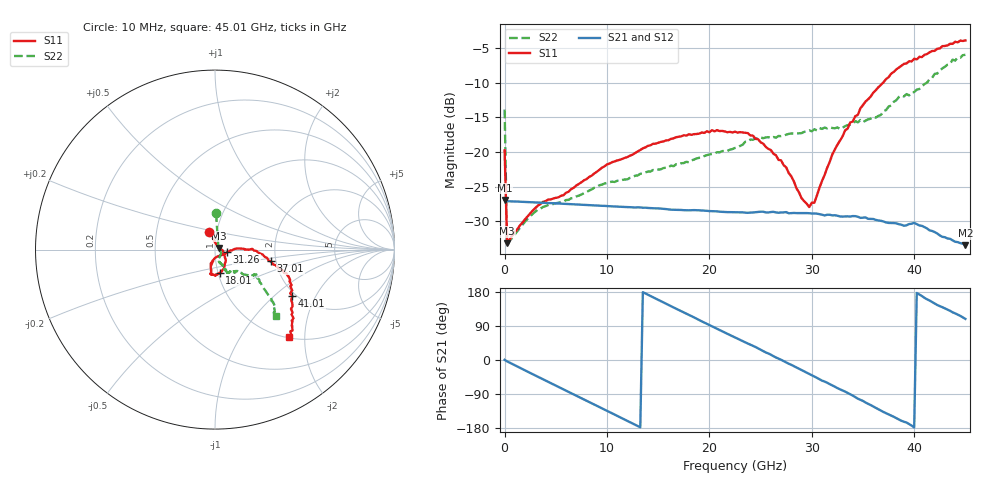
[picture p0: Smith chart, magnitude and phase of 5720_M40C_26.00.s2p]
! Device:  ADRF5720
! Description: 0.5dB LSB GaAs MMIC 6-bit Digital Attenuator
! Frequency:  0.000009 -  40 GHz
! Ports:
!	RF1	= Port 1
!	RF2	= Port 2
! Vdd:  3.3 Volt
! Vss:  -3.3 Volt
! Control:  0/3.3 Volt
! State:  26.00 dB attenuation
! Data:  The device was measured using G-S-G Probes on a matrix board.
!  Data was collected using an calibrated 4 port network analyzer.
!  The reference plane for this measurement is at the launchers.
! Note:  Analog Devices supplies this data as a sample of measured data
!  for this product.  Your particular data for this product may vary.
!  Data was taken at -40 degrees C.
!  Analog Devices reserves the right to change this data at anytime.
# GHZ S DB R 45.0
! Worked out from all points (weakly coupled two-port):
!   181 points, 10 MHz to 45.01 GHz, reference 45 ohm
!   highest |S21| = -26.90 dB at 10 MHz (marker M1); lowest = -33.4 dB at 45.01 GHz (marker M2)
!   lowest |S11| = -33.2 dB at 260 MHz (marker M3), VSWR 1.04, Z = 46.8 + j0.914 ohm
!   |S11| at or under -10 dB: start of sweep to 36.98 GHz
!   |S22| runs from -33.6 to -6.0 dB; largest |S21 - S12| = 0.0002
!   S11 on the Smith chart (normalised r, x): 10 MHz: 0.92, +0.18; 18.01 GHz: 1.02, -0.27; 31.26 GHz: 1.14, -0.03; 37.01 GHz: 1.88, -0.27; 41.01 GHz: 1.91, -1.33; 45.01 GHz: 1.02, -1.67
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0.01  -19.75 109.5  -26.90 0.4  -26.91 0.3  -13.87 88.4
0.26  -33.17 26.4  -27.08 -3.7  -27.10 -3.7  -33.56 23.0
3.26  -27.70 -4.7  -27.27 -44.3  -27.29 -44.3  -28.29 -28.6
7.76  -24.06 -32.4  -27.60 -104.2  -27.62 -104.2  -25.92 -62.1
10.01  -21.78 -43.1  -27.78 -134.2  -27.80 -134.2  -24.44 -68.3
15.26  -18.53 -66.9  -28.14 155.1  -28.16 155.1  -22.47 -70.5
18.01  -17.43 -78.9  -28.39 119.0  -28.41 119.0  -21.48 -67.2
22.76  -17.19 -99.0  -28.68 56.4  -28.70 56.3  -19.28 -65.2
24.26  -17.62 -100.1  -28.70 37.5  -28.72 37.4  -18.22 -63.4
26.01  -19.70 -103.6  -28.64 14.0  -28.66 13.9  -17.98 -62.6
27.51  -22.20 -101.8  -28.65 -6.7  -28.67 -6.9  -17.48 -63.2
29.01  -26.65 -90.4  -28.79 -26.4  -28.83 -26.5  -17.26 -63.1
29.76  -27.92 -63.5  -28.81 -36.8  -28.85 -36.9  -16.88 -63.0
30.26  -27.30 -42.5  -28.85 -43.4  -28.88 -43.5  -16.70 -61.9
31.26  -23.31 -11.5  -29.13 -56.8  -29.17 -56.9  -16.46 -58.7
33.26  -16.88 2.3  -29.27 -83.3  -29.30 -83.5  -16.25 -53.2
37.01  -9.95 -11.8  -30.00 -137.2  -30.03 -137.2  -14.09 -41.2
37.76  -8.69 -16.1  -30.22 -146.4  -30.27 -146.6  -13.28 -40.0
39.76  -6.92 -23.0  -30.32 -173.1  -30.33 -173.1  -11.40 -31.0
41.01  -5.97 -31.0  -30.82 164.1  -30.85 164.2  -10.19 -36.3
43.76  -4.39 -44.5  -32.72 125.8  -32.75 125.8  -6.67 -43.6
45.01  -3.90 -49.7  -33.41 108.4  -33.44 108.5  -5.97 -47.4
